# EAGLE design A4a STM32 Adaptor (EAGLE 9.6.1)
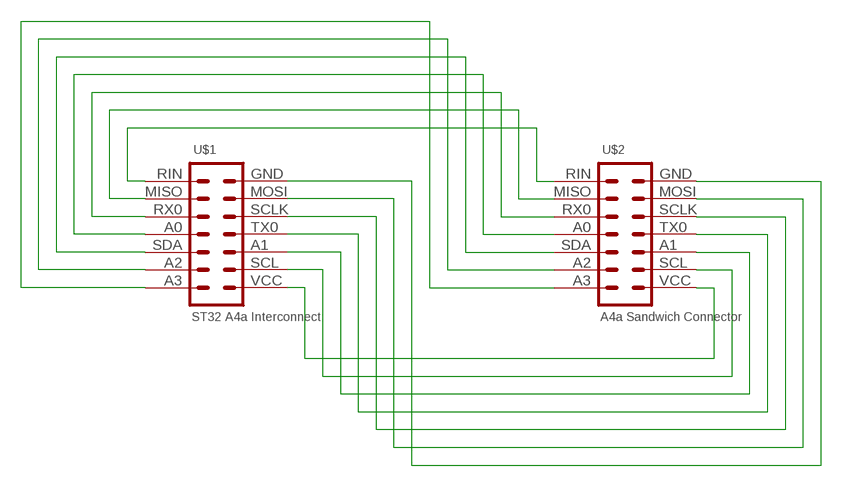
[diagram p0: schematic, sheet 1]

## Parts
U$1  ST32 A4a Interconnect  HEADER-3X5-ALF4ALL-STM32-INTERCONNECT-B  [CONN_3X5-ALF4ALL-STM32-INTERCONNECT-B]
U$2  A4a Sandwich Connector  HEADER-2X7-ALF4ALL-PROCESSOR-B  [CONN_2X7-ALF4ALL-PROCESSOR-B]

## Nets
GND: U$1.GND U$2.GND
N$1: U$1.RIN U$2.RIN
N$2: U$1.MISO U$2.MISO
N$3: U$1.RX0 U$2.RX0
N$4: U$1.A3 U$2.A3
N$5: U$1.A2 U$2.A2
N$6: U$1.SDA U$2.SDA
N$7: U$1.A0 U$2.A0
N$9: U$1.SCL U$2.SCL
N$10: U$1.A1 U$2.A1
N$11: U$1.TX0 U$2.TX0
N$12: U$1.SCLK U$2.SCLK
N$13: U$1.MOSI U$2.MOSI
VCC: U$1.VCC U$2.VCC

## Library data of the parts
U$1 = digitalconcepts:HEADER-3X5-ALF4ALL-STM32-INTERCONNECT-B: ALF4all 'Sandwich' STM32 Interconnect 3x5 Pin Header Header soldered to bottom side of PCB
U$2 = digitalconcepts:HEADER-2X7-ALF4ALL-PROCESSOR-B: ALF4all 'Sandwich' Processor (Bottom) 2x7 Pin Header Header soldered to underside of PCB

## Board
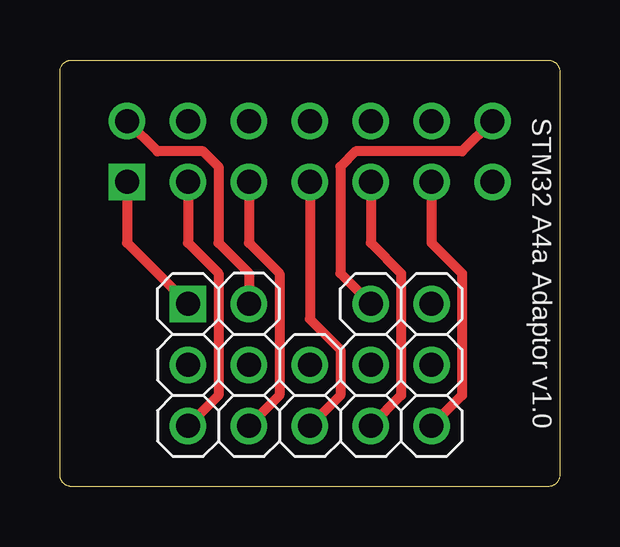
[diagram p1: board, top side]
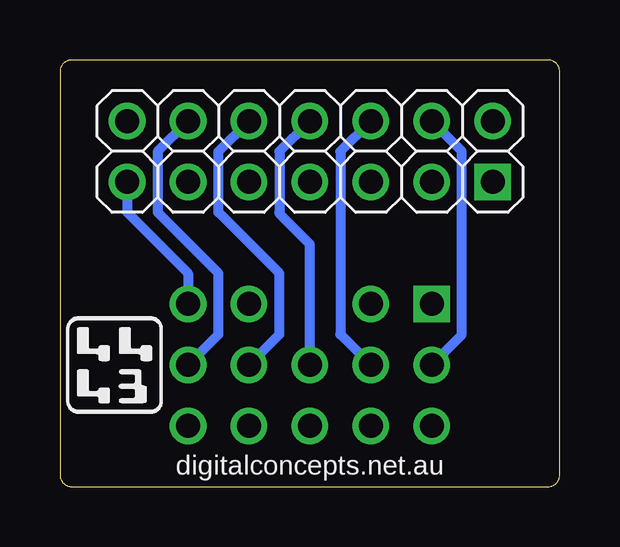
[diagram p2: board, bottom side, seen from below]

Size 20.84 x 17.78 mm. Coordinates in mm from the lower left corner, seen from the top.
Outline: 90 segments
Copper layers (1*16): Top 0.035mm / dielectric 1.5mm / Bottom 0.035mm
Design rules "default *": minimum track width 6mil, minimum drill 0.35mm, track to track 6mil, track to pad 6mil, pad to pad 6mil, via to via 6mil, smd to smd 6mil, copper to edge 6mil, drill to drill 6mil, minimum pad ring 10mil, minimum via ring 8mil, stop-mask expansion 4mil, vias tented up to drill 0mil, thermal gap 10mil

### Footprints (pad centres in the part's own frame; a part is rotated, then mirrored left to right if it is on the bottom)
CONN_3X5-ALF4ALL-STM32-INTERCONNECT-B = drill 1 pad 1.524: A0 5.08,-2.54; A1 2.54,-5.08; A2 0,-2.54; A3 2.54,0; GND 10.16,0; MISO 10.16,-2.54; MOSI 10.16,-5.08; RIN 7.62,0; RX0 7.62,-2.54; SCL 0,-5.08; SCLK 7.62,-5.08; SDA 2.54,-2.54; TX0 5.08,-5.08 | drill 1 pad 1.524 square: VCC 0,0
CONN_2X7-ALF4ALL-PROCESSOR-B = drill 1 pad 1.524: A0 7.62,2.54; A1 5.08,0; A2 2.54,2.54; A3 0,2.54; GND 15.24,0; MISO 12.7,2.54; MOSI 12.7,0; RIN 15.24,2.54; RX0 10.16,2.54; SCL 2.54,0; SCLK 10.16,0; SDA 5.08,2.54; TX0 7.62,0 | drill 1 pad 1.524 square: VCC 0,0

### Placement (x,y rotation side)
U$1  5.34,7.62 0 top
U$2  2.8,12.7 0 top

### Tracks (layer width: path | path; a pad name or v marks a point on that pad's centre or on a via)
GND
  Bottom 0.406: U$2.GND 18.04,11.43 15.5,8.89 U$1.GND
N$1
  Top 0.406: U$2.RIN 16.77,13.97 12.32,13.97 11.69,13.33 11.69,8.89 U$1.RIN
N$2
  Bottom 0.406: U$2.MISO 16.77,13.97 16.77,11.43 14.23,8.89 14.23,6.35 U$1.MISO
N$3
  Bottom 0.406: U$2.RX0 14.23,13.97 14.23,11.43 11.69,8.89 11.69,6.35 U$1.RX0
N$4
  Top 0.406: U$2.A3 4.07,13.97 5.97,13.97 6.61,13.33 6.61,10.16 7.88,8.89 U$1.A3
N$5
  Bottom 0.406: U$2.A2 4.11,14 4.11,6.31 U$1.A2
N$6
  Bottom 0.406: U$2.SDA 9.15,13.97 9.15,6.35 U$1.SDA
N$7
  Bottom 0.406: U$1.A0 10.42,10.1 11.67,11.35 11.69,11.43 11.69,13.97 U$2.A0
N$9
  Top 0.406: U$2.SCL 5.34,10.16 6.61,8.89 6.61,3.81 U$1.SCL
N$10
  Top 0.406: U$2.A1 7.88,10.16 9.15,8.89 9.15,3.81 U$1.A1
N$11
  Top 0.406: U$2.TX0 10.42,6.98 11.69,5.71 11.69,3.81 U$1.TX0
N$12
  Top 0.406: U$2.SCLK 12.96,10.16 14.23,8.89 14.23,3.81 U$1.SCLK
N$13
  Top 0.406: U$2.MOSI 15.5,10.16 16.77,8.89 16.77,3.81 U$1.MOSI
VCC
  Top 0.406: U$2.VCC 2.8,10.16 U$1.VCC

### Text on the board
tPlace: STM32 A4a Adaptor v1.0
bPlace: digitalconcepts.net.au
